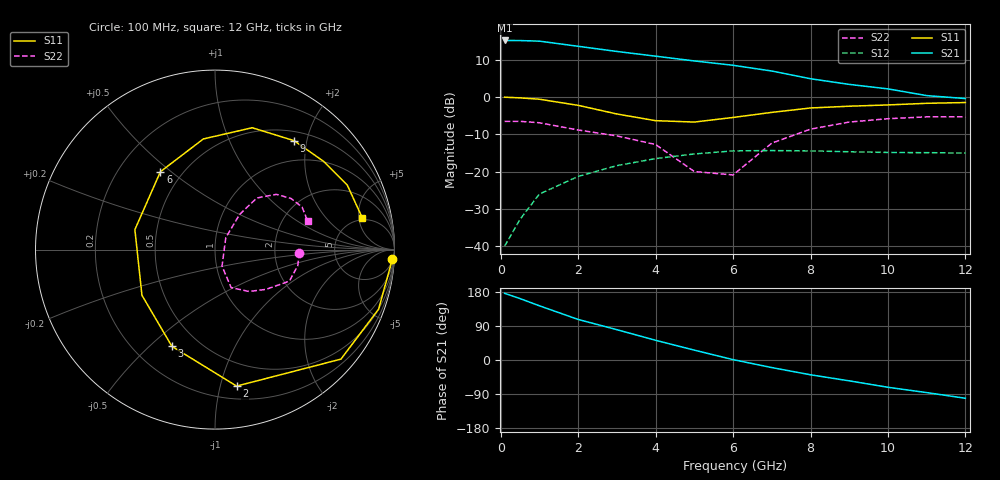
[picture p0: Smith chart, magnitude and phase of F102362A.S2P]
!ATF-10236
!S-PARAMETERS at Vds=2V  Id=25mA.  LAST UPDATED 06-27-94
# ghz s ma r 50
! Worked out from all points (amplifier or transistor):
!   14 points, 100 MHz to 12 GHz, reference 50 ohm
!   highest |S21| = 15.1 dB at 100 MHz (marker M1)
!   |S21| within 3 dB of that: start of sweep to 3.042 GHz
!   unconditionally stable (mu >= 1): 5.33 GHz to end of sweep
!   at 1 GHz: K = 0.27, MSG = 20.5 dB, |S12| = -26.0 dB
!   at 6 GHz: K = 1.01, MAG = 10.9 dB, |S12| = -14.5 dB
!   at 12 GHz: K = 1.09, MAG = 5.5 dB, |S12| = -15.0 dB
!   lowest NFmin = 0.40 dB at 500 MHz
!   S11 on the Smith chart (normalised r, x): 100 MHz: 7, -37; 2 GHz: 0.30, -1.13; 3 GHz: 0.36, -0.59; 6 GHz: 0.38, +0.46; 9 GHz: 0.64, +1.78; 12 GHz: 4.72, +5.61
0.1  0.99 -3.0  5.7 176.0  0.01 74.0  0.47 -2.0
0.5  0.97 -20.0  5.68 162.0  0.023 76.0  0.47 -11.0
1  0.93 -41.0  5.58 143.0  0.05 71.0  0.45 -23.0
2  0.77 -81.0  4.76 107.0  0.086 51.0  0.36 -38.0
3  0.59 -114.0  4.06 80.0  0.12 35.0  0.3 -51.0
4  0.48 -148.0  3.51 52.0  0.149 18.0  0.23 -67.0
5  0.46 166.0  3.03 26.0  0.172 3.0  0.1 -67.0
6  0.53 125.0  2.65 1.0  0.189 -14.0  0.09 48.0
7  0.62 96.0  2.22 -20.0  0.191 -28.0  0.24 55.0
8  0.71 73.0  1.75 -39.0  0.189 -41.0  0.37 51.0
9  0.75 54.0  1.47 -55.0  0.184 -46.0  0.46 42.0
10  0.78 39.0  1.28 -72.0  0.18 -59.0  0.51 34.0
11  0.82 26.0  1.04 -86.0  0.179 -71.0  0.54 26.0
12  0.84 12.0  0.95 -101.0  0.177 -82.0  0.54 17.0
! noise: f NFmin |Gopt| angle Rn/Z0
0.5  0.4  0.94  16  0.78
1  0.5  0.87  36  0.63
2  0.6  0.73  74  0.33
4  0.8  0.45  148  0.15
6  1  0.42  -137  0.12
8  1.3  0.49  -80  0.45
12  1.6  0.65  -20  1.16
